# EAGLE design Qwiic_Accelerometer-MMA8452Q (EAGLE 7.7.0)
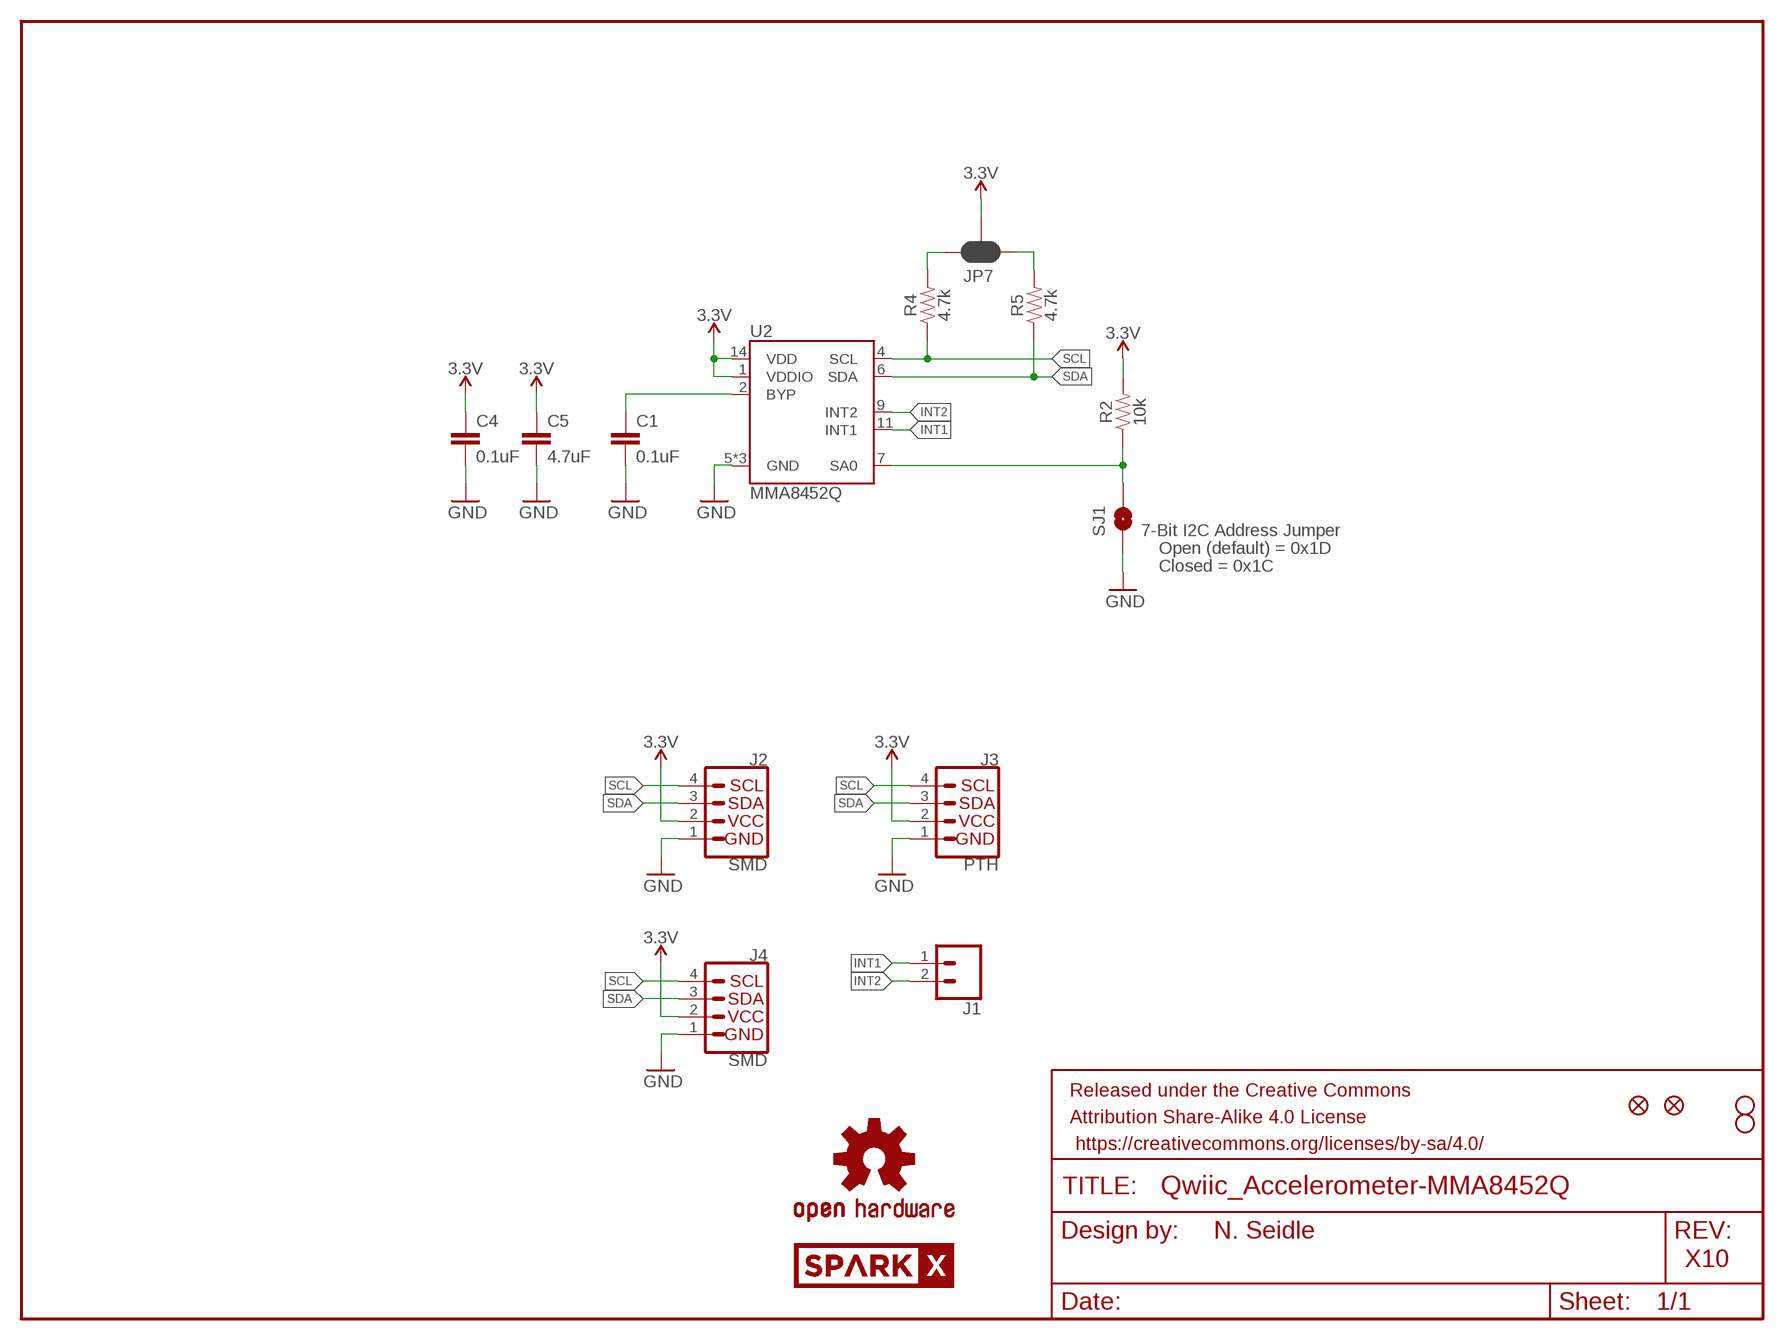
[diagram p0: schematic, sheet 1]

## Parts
C1  0.1uF  0.1UF-0603-25V-(+80/-20%)  [0603]
C4  0.1uF  0.1UF-0603-25V-(+80/-20%)  [0603]
C5  4.7uF  4.7UF0603  [0603]
FRAME1  FRAME-LETTER  [CREATIVE_COMMONS]
J1  CONN_021X02_NO_SILK  [1X02_NO_SILK]
J2  SMD  I2C_STANDARDJS-1MM  [1X04_1MM_RA]
J3  PTH  I2C_STANDARD_NO_SILK  [1X04_NO_SILK]
J4  SMD  I2C_STANDARDJS-1MM  [1X04_1MM_RA]
JP2  FIDUCIALUFIDUCIAL  [MICRO-FIDUCIAL]
JP3  STAND-OFF  [STAND-OFF]
JP4  STAND-OFF  [STAND-OFF]
JP6  FIDUCIALUFIDUCIAL  [MICRO-FIDUCIAL]
JP7  JUMPER-SMT_3_2-NC_PASTE_SILK  [SMT-JUMPER_3_2-NC_PASTE_SILK]
LOGO1  OSHW-LOGOMINI  [OSHW-LOGO-MINI]
R2  10k  10KOHM-0603-1/10W-1%  [0603]
R4  4.7k  4.7KOHM-0603-1/10W-1%  [0603]
R5  4.7k  4.7KOHM-0603-1/10W-1%  [0603]
SJ1  SOLDERJUMPERNO  [SJ_2S-NO]
U2  MMA8452Q  [QFN-16_0.5MM]
U$1  SPARKX-LOGO4  [SPARKX-MEDIUM]
U$2  SPARKX-LOGO4  [SPARKX-MEDIUM]

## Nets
3.3V: C4.1 C5.1 J2.2(VCC) J3.2(VCC) J4.2(VCC) JP7.2 R2.2 U2.1(VDDIO) U2.14(VDD)
BYP: C1.1 U2.2(BYP)
GND: C1.2 C4.2 C5.2 J2.1(GND) J3.1(GND) J4.1(GND) SJ1.1 U2.5(GND) U2.10(GND) U2.12(GND)
INT1: J1.1 U2.11(INT1)
INT2: J1.2 U2.9(INT2)
N$1: JP7.1 R5.2
N$2: JP7.3 R4.2
SA0: R2.1 SJ1.2 U2.7(SA0)
SCL: J2.4(SCL) J3.4(SCL) J4.4(SCL) R4.1 U2.4(SCL)
SDA: J2.3(SDA) J3.3(SDA) J4.3(SDA) R5.1 U2.6(SDA)

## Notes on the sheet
- 7-Bit I2C Address Jumper
- Open (default) = 0x1D
- Closed = 0x1C
- N. Seidle
- X10

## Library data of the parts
C1 C4 = SparkFun-Capacitors:0.1UF: 0.1µF ceramic capacitors; PROD_ID: CAP-00810
C5 = SparkFun-Capacitors:4.7UF: 4.7µF ceramic capacitors; PROD_ID: CAP-08280
FRAME1 = SparkFun-Aesthetics:FRAME-LETTER: Schematic Frame - Letter
J1 = SparkFun-Connectors:CONN_02: Multi connection point. Often used as Generic Header-pin footprint for 0.1 inch spaced/style header connections
J2-J4 = SparkX:I2C_STANDARD: SparkFun I2C Standard Pinout Header SparkFun has standardized on a pinout for all I2C based sensor breakouts. This pinout allows I2C boards to be plugged directly into the headers on Arduino Uno compatible boards, and to be daisy chained easily. Example SparkFun Products: SparkFun Atmospheric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
JP2 JP6 = SparkFun:FIDUCIAL: Fiducial Alignment Points
JP3 JP4 = SparkFun:STAND-OFF: Stand Off
JP7 = SparkFun-Jumpers:JUMPER-SMT_3_2-NC_PASTE: Normally closed solder jumper (2 of 2 connections) This jumper has an aperture in the stencil to allow solder paste to bridge both connections. Both connections are normally closed (NC). Wick off the solder to open the connection(s). Reapply solder to reclose the connection(s).
LOGO1 = SparkFun-Aesthetics:OSHW-LOGO: Open-Source Hardware (OSHW) Logo
R2 = SparkFun-Resistors:10KOHM: 10kΩ resistor; PROD_ID: RES-00824
R4 R5 = SparkFun-Resistors:4.7KOHM: 4.7kΩ resistor; PROD_ID: RES-07857
SJ1 = SparkFun:SOLDERJUMPER: Solder Jumper
U2 = SparkX:MMA8452Q: MMA8452Q 3-Axis, 12/8-bit Digital Accelerometer Supply Voltage: 1.6-3.6V Range: +/- 2g, 4g, 8g Interface: I2C, 12-bit and 8-bit ODR: 1.56 Hz - 800 Hz Package: QFN-16 http://cache.freescale.com/files/sensors/doc/data_sheet/MMA8452Q.pdf
U$1 U$2 = SparkX:SPARKX-LOGO

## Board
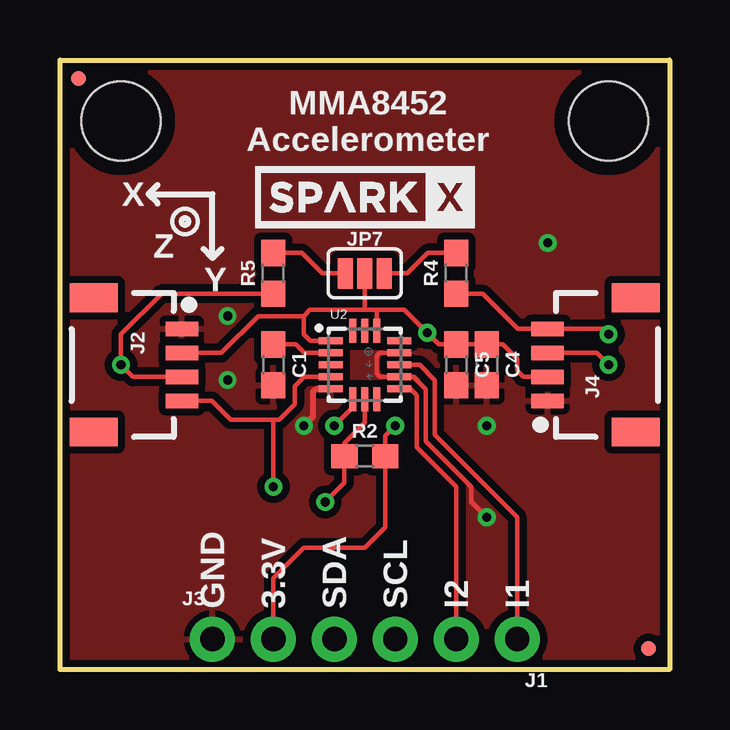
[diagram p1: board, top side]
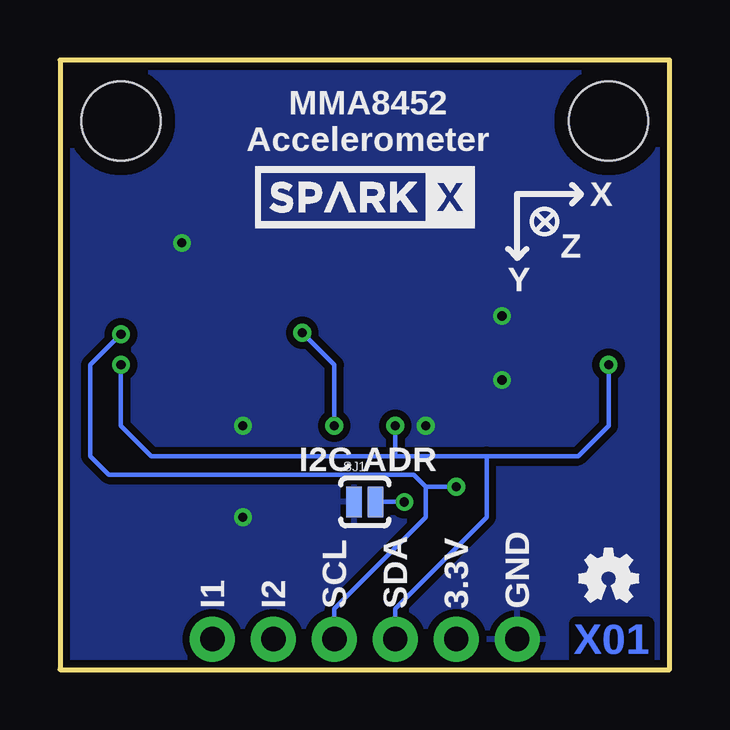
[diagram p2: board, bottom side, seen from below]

Size 25.4 x 25.4 mm. Coordinates in mm from the lower left corner, seen from the top.
Outline: 0,0 0,25.4 25.4,25.4 25.4,0 0,0
Copper layers (1*16): Top 0.035mm / dielectric 1.5mm / Bottom 0.035mm
Design rules "SparkFun-2-layer-TIGHT": minimum track width 7mil, minimum drill 15mil, track to track 7mil, track to pad 7mil, pad to pad 7mil, via to via 7mil, smd to smd 7mil, copper to edge 7mil, drill to drill 7mil, minimum pad ring 7mil, minimum via ring 7mil, stop-mask expansion 4mil, vias tented up to drill 25mil, thermal gap 10mil

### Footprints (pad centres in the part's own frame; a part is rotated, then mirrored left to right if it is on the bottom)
0603 = smd 1.1 x 1: 1 -0.85,0; 2 0.85,0
1X02_NO_SILK = drill 1.016 pad 1.88: 1 0,0; 2 2.54,0
1X04_1MM_RA = smd 0.6 x 1.35: 1 -1.5,0; 2 -0.5,0; 3 0.5,0; 4 1.5,0 | smd 1.2 x 2: NC1 2.8,-3.675; NC2 -2.8,-3.675
1X04_NO_SILK = drill 1.016 pad 1.88: 1 0,0; 2 2.54,0; 3 5.08,0; 4 7.62,0
MICRO-FIDUCIAL = smd 0.635 x 0.635: 1 0,0
STAND-OFF = hole 3.302: 0,0
SMT-JUMPER_3_2-NC_PASTE_SILK = smd 0.635 x 1.27: 1 -0.813,0; 2 0,0; 3 0.813,0
SJ_2S-NO = smd 0.635 x 1.27: 1 -0.45,0; 2 0.45,0
QFN-16_0.5MM = smd 1 x 0.3: 1 -1.425,1; 2 -1.425,0.5; 3 -1.425,0; 4 -1.425,-0.5; 5 -1.425,-1; 9 1.425,-1; 10 1.425,-0.5; 11 1.425,0; 12 1.425,0.5; 13 1.425,1 | smd 0.3 x 1: 6 -0.5,-1.425; 7 0,-1.425; 8 0.5,-1.425; 14 0.5,1.425; 15 0,1.425; 16 -0.5,1.425

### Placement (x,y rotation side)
C1  8.89,12.7 270 top
C4  17.78,12.7 270 top
C5  16.51,12.7 270 top
FRAME1  not placed on the board
J1  19.05,1.27 180 top
J2  5.08,12.7 270 top
J3  6.35,1.27 0 top
J4  20.32,12.7 90 top
JP2  24.51,0.89 0 top
JP3  2.54,22.86 0 top
JP4  22.86,22.86 0 top
JP6  0.76,24.64 0 top
JP7  12.7,16.51 0 top
LOGO1  2.54,3.81 0 bottom
R2  12.7,8.89 0 top
R4  16.51,16.51 90 top
R5  8.89,16.51 90 top
SJ1  12.7,6.99 0 bottom
U2  12.7,12.7 0 top
U$1  12.7,19.68 0 bottom
U$2  12.7,19.68 0 top

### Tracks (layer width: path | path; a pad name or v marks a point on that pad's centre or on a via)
3.3V  (via drill 0.38)
  Top 0.178: J4.2 19.3,12.2 19.05,12.45 19.05,12.95 18.45,13.55 C4.1 C5.1 15.79,13.55 v15.3,14.03 14.35,14.99 13.21,14.99 | 10.16,14.73 8.26,14.73 6.72,13.2 J2.2 | U2.1 10.43,13.7 10.16,13.97 10.16,14.73 | v13.97,10.16 13.55,9.74 R2.2 13.55,5.93 12.7,5.08 10.16,5.08 8.89,3.81 J3.2 | 13.21,14.99 12.7,14.99 | 12.7,14.99 10.41,14.99 10.16,14.73 | U2.14 13.2,14.98 13.21,14.99 | JP7.2 12.7,14.99
  Bottom 0.178: v13.97,10.16 13.97,12.7 v15.3,14.03
BYP
  Top 0.178: U2.2 10.17,13.2 9.82,13.55 C1.1
GND  (via drill 0.38)
  Top 0.178: v17.78,6.35 17.14,6.99 17.14,7.62 15.24,9.53 15.24,11.68 14.72,12.2 U2.10 13.33,12.2 13.21,12.32 13.21,13.08 13.33,13.2 U2.12
  Top 0.254: U2.5 10.68,11.7 10.54,11.56 10.54,10.54 v10.16,10.16
  other vias: 6.99,12.06 6.99,14.73 17.78,10.16 20.32,17.78
  pour Bottom (isolate 0.305): 0,0 0,25.4 25.4,25.4 25.4,0
  pour Top (isolate 0.305): 0,0 0,25.4 25.4,25.4 25.4,0
INT1
  Top 0.178: U2.11 14.99,12.7 15.62,12.06 15.62,9.78 19.05,6.35 J1.1
INT2
  Top 0.178: U2.9 14.59,11.7 14.86,11.43 14.86,9.27 16.51,7.62 J1.2
N$1
  Top 0.178: JP7.1 10.92,16.51 10.07,17.36 R5.2
N$2
  Top 0.178: JP7.3 14.48,16.51 15.33,17.36 R4.2
SA0  (via drill 0.38)
  Top 0.178: U2.7 12.7,10.29 11.85,9.44 R2.1 11.85,7.79 v11.05,6.99
  Bottom 0.178: SJ1.2 v11.05,6.99
SCL  (via drill 0.38)
  Top 0.178: R4.1 17.61,15.66 19.07,14.2 J4.4 22.63,14.2 v22.86,13.97 | U2.4 10.17,12.2 9.78,11.81 9.78,11.05 9.14,10.41 8.89,10.41 | 8.89,10.41 7.11,10.41 6.33,11.2 J2.4 | 8.89,10.41 v8.89,7.62
  Bottom 0.178: v22.86,13.97 24.13,12.7 24.13,8.89 23.37,8.13 10.67,8.13 10.16,7.62 | J3.4 13.97,2.54 10.16,6.35 10.16,7.62 | 10.16,7.62 v8.89,7.62
SDA  (via drill 0.38)
  Top 0.178: U2.6 12.2,10.93 v11.43,10.16 | J4.3 22.36,13.2 v22.86,12.7 | J2.3 3.04,12.2 v2.54,12.7 2.54,13.97 4.23,15.66 R5.1
  Bottom 0.178: v22.86,12.7 22.86,10.16 21.59,8.89 11.43,8.89 | 11.43,8.89 7.62,8.89 | 7.62,8.89 3.81,8.89 2.54,10.16 v2.54,12.7 | J3.3 11.43,2.54 7.62,6.35 7.62,8.89 | v11.43,10.16 11.43,8.89

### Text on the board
Bottom: X01
tPlace: MMA8452 / Accelerometer | X | Z | Y | GND | 3.3V | SDA | SCL | I2 | I1
bPlace: MMA8452 / Accelerometer | X | Z | Y | I2C ADR | GND | 3.3V | SDA | SCL | I2 | I1

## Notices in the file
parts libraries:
SparkFun-Resistors: Licensing: Creative Commons ShareAlike 4.0 International - https://creativecommons.org/licenses/by-sa/4.0
SparkFun-Aesthetics: Released under the Creative Commons Attribution Share-Alike 4.0 License
SparkFun-Aesthetics: https://creativecommons.org/licenses/by-sa/4.0
